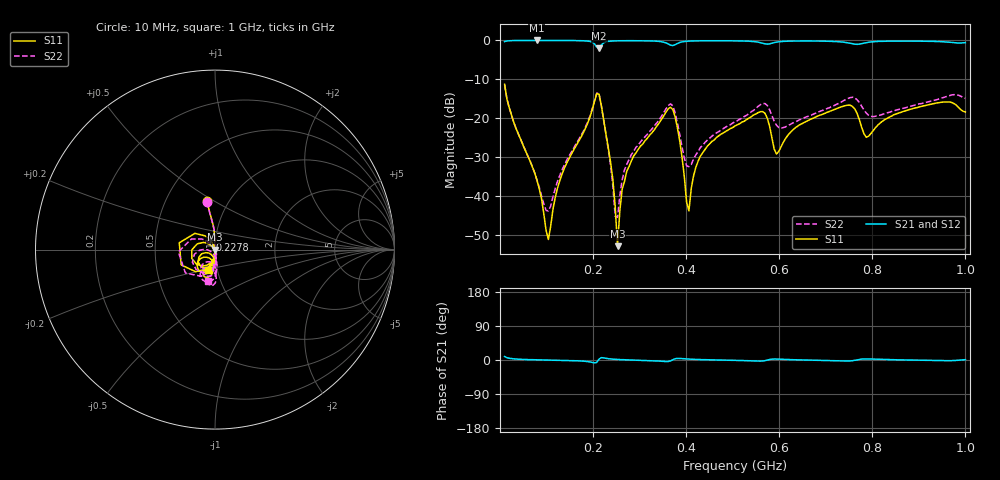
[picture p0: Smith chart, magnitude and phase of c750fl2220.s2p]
!Agilent Technologies,N5234A,MY52241123,A.10.00.00
!Agilent N5234A: A.10.00.00
!Date: Friday, January 04, 2019 08:25:31
!Correction: S11(Full 2 Port(1,2))
!S21(Full 2 Port(1,2))
!S12(Full 2 Port(1,2))
!S22(Full 2 Port(1,2))
!S2P File: Measurements: S11, S21, S12, S22:
# Hz S  dB  R 50
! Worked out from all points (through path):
!   201 points, 10 MHz to 1 GHz, reference 50 ohm
!   highest |S21| = -0.01 dB at 79.3 MHz (marker M1); lowest = -2.1 dB at 212.9 MHz (marker M2)
!   lowest |S11| = -52.9 dB at 252.6 MHz (marker M3), VSWR 1.00, Z = 49.8 - j0.0334 ohm
!   |S11| at or under -10 dB: start of sweep to end of sweep
!   |S22| runs from -45.5 to -11.4 dB; largest |S21 - S12| = 0.0045
!   S11 on the Smith chart (normalised r, x): 10 MHz: 0.79, +0.46; 227.8 MHz: 0.94, +0.10; 1 GHz: 0.90, -0.21
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1e7  -11.28 99.6  -0.31 9.1  -0.30 9.3  -11.40 100.0
7.93e7  -35.89 81.4  -0.01 0.5  -0.01 0.4  -35.88 73.5
1.0405e8  -51.24 -4.2  -0.01 -0.1  -0.01 -0.2  -43.88 -6.1
1.288e8  -36.01 -81.8  -0.02 -0.7  -0.02 -0.7  -34.66 -65.8
1.783e8  -23.95 -99.6  -0.09 -2.9  -0.09 -3.0  -23.60 -86.3
2.1295e8  -13.86 169.2  -2.07 2.4  -2.07 2.4  -13.78 -176.5
2.278e8  -24.09 117.0  -0.37 4.4  -0.37 4.4  -24.32 132.9
2.4265e8  -35.91 109.6  -0.14 2.2  -0.15 2.2  -37.54 133.9
2.5255e8  -52.94 -171.4  -0.10 1.4  -0.10 1.5  -45.53 -110.9
2.7235e8  -33.70 -93.1  -0.08 0.4  -0.08 0.4  -31.93 -79.0
3.4165e8  -21.29 -112.4  -0.25 -2.9  -0.25 -2.9  -20.51 -92.1
3.7135e8  -17.76 -179.2  -1.34 0.6  -1.35 0.7  -16.83 -150.9
4.06e8  -43.85 -129.8  -0.19 2.4  -0.19 2.4  -32.47 -127.9
4.3075e8  -29.75 -88.5  -0.10 1.1  -0.10 1.2  -27.53 -89.2
5.05e8  -22.01 -97.3  -0.12 -0.9  -0.12 -0.9  -20.97 -82.7
5.644e8  -18.31 -134.0  -0.73 -2.7  -0.72 -2.7  -16.25 -105.0
5.941e8  -29.22 -131.1  -0.45 2.4  -0.45 2.4  -21.80 -123.2
6.733e8  -20.00 -97.0  -0.16 -0.5  -0.17 -0.5  -18.99 -88.1
7.525e8  -16.67 -127.3  -0.74 -2.5  -0.75 -2.5  -14.73 -102.5
7.8715e8  -24.94 -123.9  -0.57 2.9  -0.57 2.9  -18.71 -118.8
8.3665e8  -19.72 -93.5  -0.19 1.0  -0.20 0.9  -18.47 -93.2
1e9  -18.41 -108.5  -0.56 0.9  -0.56 0.8  -14.95 -101.8
